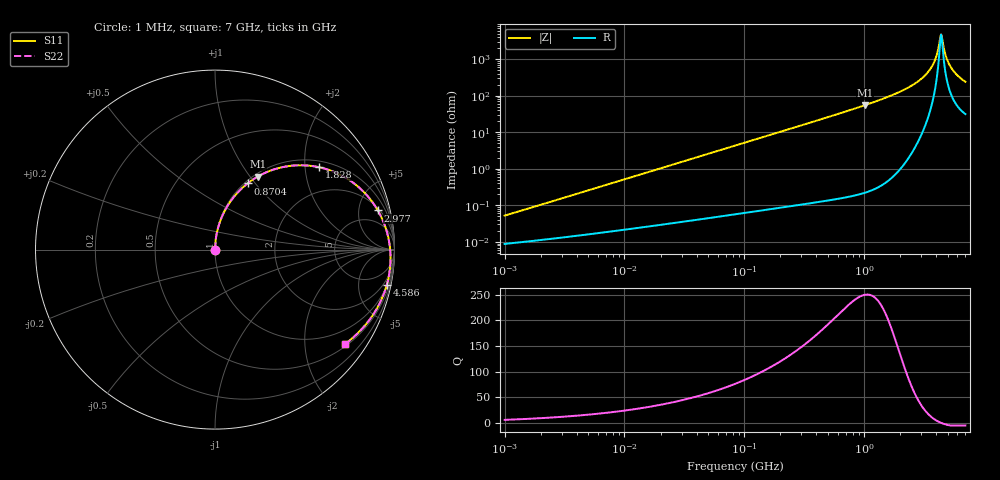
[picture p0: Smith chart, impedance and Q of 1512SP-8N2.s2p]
# MHz  S  MA  R  50
!Freq  MagS11  AngS11  MagS21  AngS21  MagS12  AngS12  MagS22  AngS22
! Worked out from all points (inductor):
!   801 points, 1 MHz to 7 GHz, reference 50 ohm
!   read as one part in series: L = 8.19 nH near 1.045 MHz
!   highest Q = 250 at 1.016 GHz (marker M1), where L = 8.65 nH
!   self-resonance near 4.387 GHz
!   S11 on the Smith chart (normalised r, x): 1 MHz: 1.00, +0.00; 870.4 MHz: 1.03, +0.91; 1.828 GHz: 1.17, +2.38; 2.977 GHz: 2.29, +7.77; 4.586 GHz: 1.13, -9.76; 7 GHz: 0.56, -2.99
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1  0.0005051 80.0  0.9999 -0.0  0.9999 -0.0  0.000505 80.0
4.412787  0.0022 85.9  0.9998 -0.1  0.9998 -0.1  0.0022 85.9
19.25816  0.009581 87.7  0.9997 -0.6  0.9997 -0.6  0.00958 87.7
84.04588  0.04177 86.7  0.9986 -2.6  0.9986 -2.6  0.04176 86.7
366.7906  0.1806 78.5  0.9824 -11.1  0.9824 -11.1  0.1805 78.5
870.3599  0.4109 63.8  0.91 -26.0  0.91 -26.0  0.4108 63.8
1016.382  0.4713 59.7  0.88 -30.1  0.88 -30.1  0.4712 59.7
1600.737  0.677 44.0  0.7325 -45.7  0.7325 -45.7  0.6768 44.0
1828.333  0.7405 38.3  0.6675 -51.4  0.6675 -51.4  0.7403 38.3
2332.941  0.8493 26.6  0.5183 -62.7  0.5183 -62.7  0.8491 26.6
2976.817  0.9333 13.5  0.3335 -74.8  0.3335 -74.8  0.9331 13.5
3400.069  0.9627 6.0  0.2221 -80.8  0.2221 -80.8  0.9625 6.0
3756.551  0.9756 0.2  0.1365 -83.4  0.1365 -83.4  0.9755 0.2
3970.505  0.9793 -3.1  0.08914 -82.2  0.08914 -82.2  0.9792 -3.1
4243.395  0.9803 -7.0  0.03571 -64.6  0.03571 -64.6  0.9804 -7.0
4338.465  0.9799 -8.3  0.02286 -37.6  0.02286 -37.6  0.98 -8.3
4435.664  0.9791 -9.6  0.02212 10.6  0.02212 10.6  0.9792 -9.6
4585.562  0.9772 -11.5  0.04194 46.7  0.04194 46.7  0.9773 -11.6
4900.724  0.9709 -15.5  0.09393 59.3  0.09393 59.3  0.9712 -15.5
5295.895  0.9598 -20.0  0.1548 59.5  0.1548 59.5  0.9602 -20.0
5982.236  0.9355 -27.0  0.2447 54.9  0.2447 54.9  0.9362 -27.0
7000  0.8957 -35.9  0.3454 46.9  0.3454 46.9  0.897 -35.9
